TYPE Alarm :
STRUCT
	PRESSURE:BOOL;
	MFC1:BOOL;
	MFC2:BOOL;
	MFC3:BOOL;
	MFC5:BOOL;
	MFC6:BOOL;
	MFC7:BOOL;
	WALL_TEMP:BOOL;
	LID_TEMP:BOOL;
	STAGE_EDGE_TEMP:BOOL;
	STAGE_CENTER_TEMP: BOOL;
	Gas1FlowPressureOutOfRange:BOOL;
	Gas2FlowPressureOutOfRange:BOOL;
	Gas3FlowPressureOutOfRange:BOOL;
	Gas4FlowPressureOutOfRange:BOOL;
	Gas5FlowPressureOutOfRange:BOOL;
	Gas6FlowPressureOutOfRange:BOOL;
	TurboN2PurgePressureOutOfRange:BOOL;
	PrepareTransferTimerout:BOOL;
	TransferWaferTimeout:BOOL;
	OpenGasValveTimeout:BOOL;
	CloseGasValveTimeout:BOOL;
	OpenCloseSlitValveTimeout:BOOL;
	ATMCheckTimeout:BOOL;
	
	PLC				:BOOL;	
	DRY_PUMP		:BOOL;
	PENDULUM_VALVE	:BOOL;
	TURBO_PUMP		:BOOL;
	CHILLER1		:BOOL;
	CHILLER2		:BOOL;
	
	//PROCESS TOLERANCE
	TOLERANCE_PRESSURE:BOOL;
	TOLERANCE_MFC1:BOOL;
	TOLERANCE_MFC2:BOOL;
	TOLERANCE_MFC3:BOOL;
	TOLERANCE_MFC5:BOOL;
	TOLERANCE_MFC6:BOOL;
	TOLERANCE_MFC7:BOOL;
	TOLERANCE_WALL_TEMP:BOOL;
	TOLERANCE_LID_TEMP:BOOL;
	TOLERANCE_STAGE_EDGE_TEMP:BOOL;
	TOLERANCE_STAGE_CENTER_TEMP: BOOL;
END_STRUCT
END_TYPE
